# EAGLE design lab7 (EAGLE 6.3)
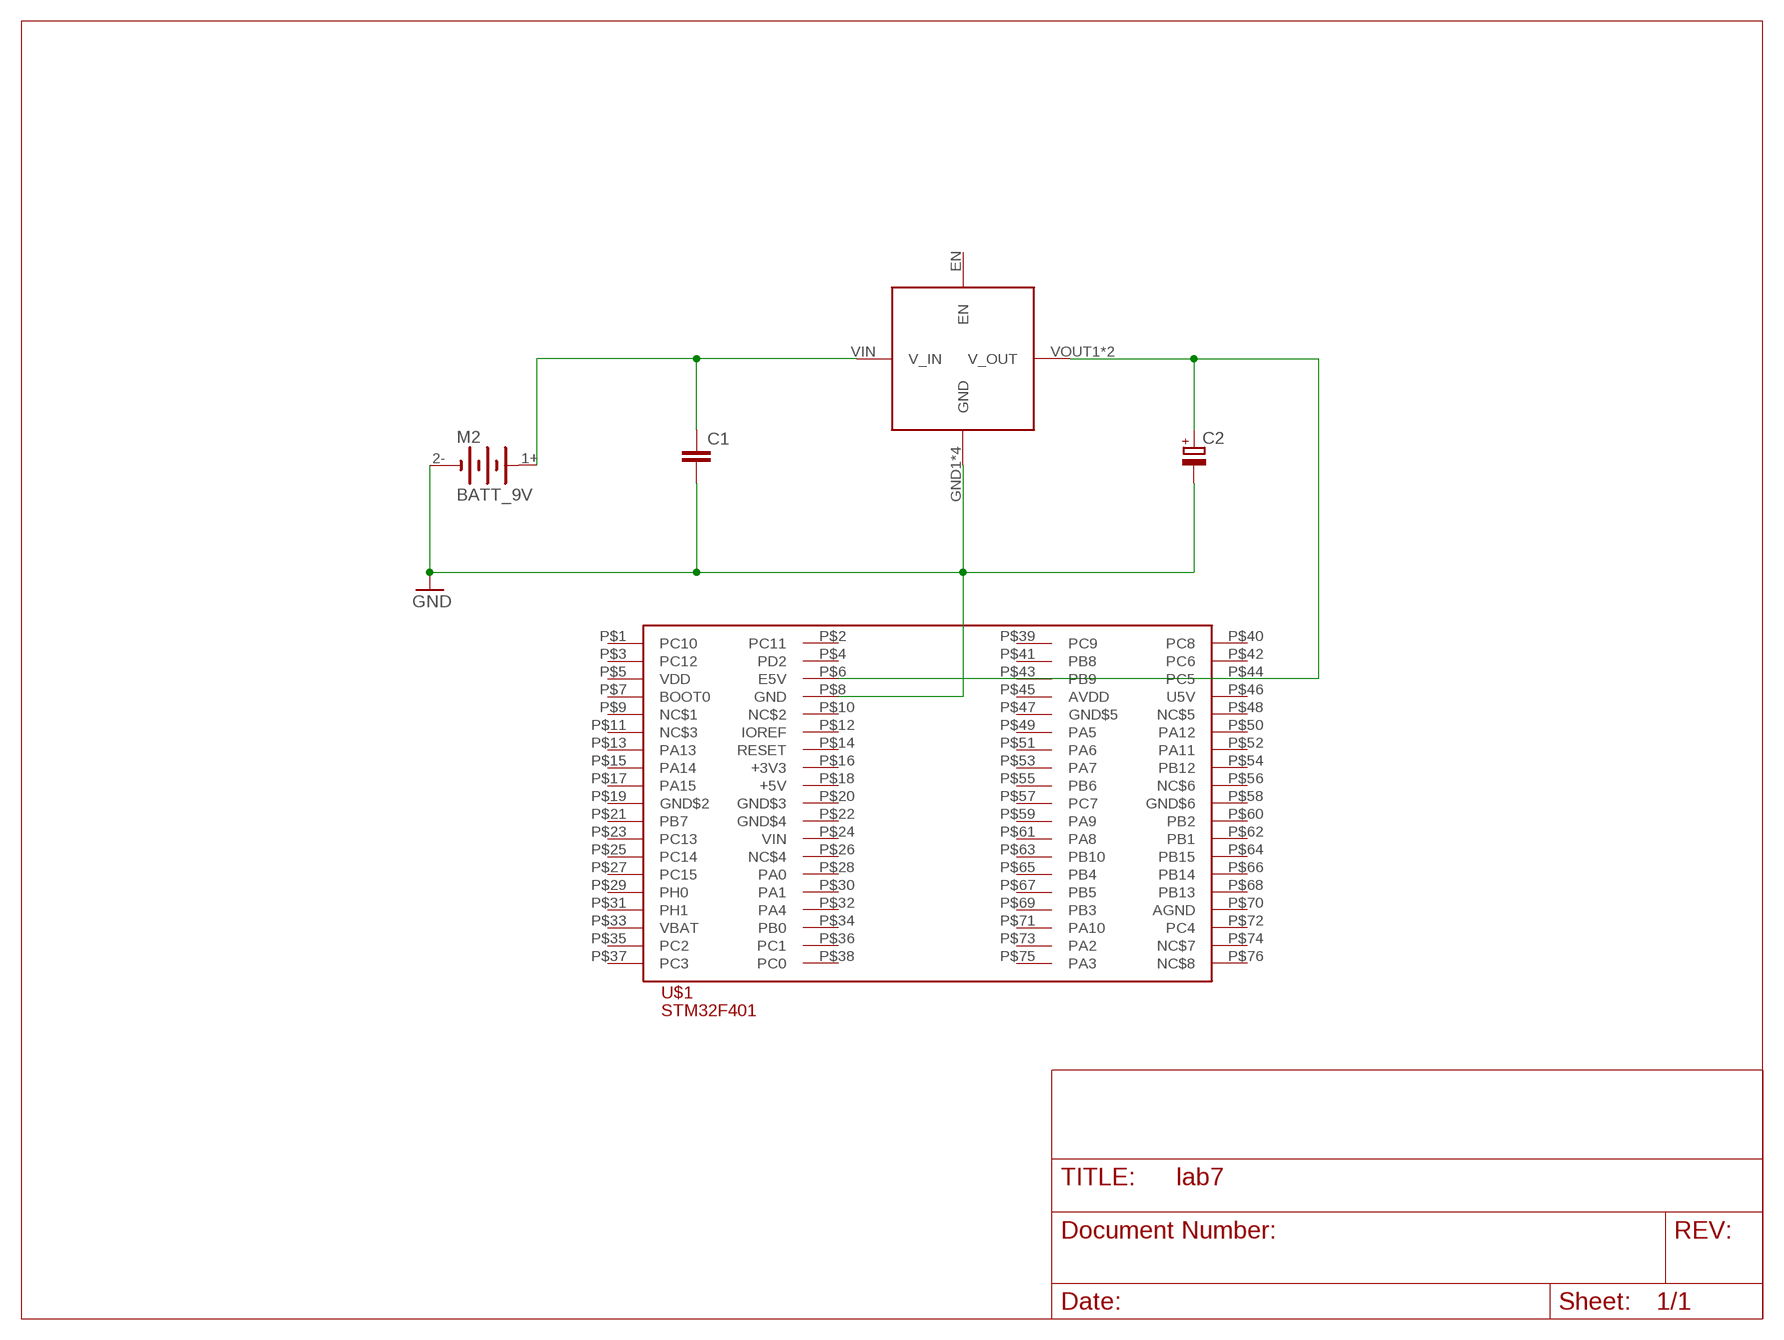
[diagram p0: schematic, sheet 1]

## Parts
C1  C-EU025-025X050  [C025-025X050]
C2  CPOL-EUE3.5-8  [E3,5-8]
M1  PWR_REG  [PWR_REG]
M2  BATT_9V  [BATT_9V]
U$1  STM32401RESTM32P38PKG  [STM32P38]

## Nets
GND: C1.2 C2.- M1.GND1(GND) M1.GND2(GND) M1.GND3(GND) M1.GND4(GND) M2.2-(-) U$1.P$8(GND)
N$2: C1.1 M1.VIN(V_IN) M2.1+(+)
N$3: C2.+ M1.VOUT1(V_OUT) M1.VOUT2(V_OUT) U$1.P$6(E5V)
Unconnected: M1.EN U$1.P$1(PC10) U$1.P$2(PC11) U$1.P$3(PC12) U$1.P$4(PD2) U$1.P$5(VDD) U$1.P$7(BOOT0) U$1.P$9(NC$1) U$1.P$10(NC$2) U$1.P$11(NC$3) U$1.P$12(IOREF) U$1.P$13(PA13) U$1.P$14(RESET) U$1.P$15(PA14) U$1.P$16(+3V3) U$1.P$17(PA15) U$1.P$18(+5V) U$1.P$19(GND$2) U$1.P$20(GND$3) U$1.P$21(PB7) U$1.P$22(GND$4) U$1.P$23(PC13) U$1.P$24(VIN) U$1.P$25(PC14) U$1.P$26(NC$4) U$1.P$27(PC15) U$1.P$28(PA0) U$1.P$29(PH0) U$1.P$30(PA1) U$1.P$31(PH1) U$1.P$32(PA4) U$1.P$33(VBAT) U$1.P$34(PB0) U$1.P$35(PC2) U$1.P$36(PC1) U$1.P$37(PC3) U$1.P$38(PC0) U$1.P$39(PC9) U$1.P$40(PC8) U$1.P$41(PB8) U$1.P$42(PC6) U$1.P$43(PB9) U$1.P$44(PC5) U$1.P$45(AVDD) U$1.P$46(U5V) U$1.P$47(GND$5) U$1.P$48(NC$5) U$1.P$49(PA5) U$1.P$50(PA12) U$1.P$51(PA6) U$1.P$52(PA11) U$1.P$53(PA7) U$1.P$54(PB12) U$1.P$55(PB6) U$1.P$56(NC$6) U$1.P$57(PC7) U$1.P$58(GND$6) U$1.P$59(PA9) U$1.P$60(PB2) U$1.P$61(PA8) U$1.P$62(PB1) U$1.P$63(PB10) U$1.P$64(PB15) U$1.P$65(PB4) U$1.P$66(PB14) U$1.P$67(PB5) U$1.P$68(PB13) U$1.P$69(PB3) U$1.P$70(AGND) U$1.P$71(PA10) U$1.P$72(PC4) U$1.P$73(PA2) U$1.P$74(NC$7) U$1.P$75(PA3) U$1.P$76(NC$8)

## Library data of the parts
C1 = rcl:C-EU: CAPACITOR, European symbol
C2 = rcl:CPOL-EU: POLARIZED CAPACITOR, European symbol
M1 = P442:PWR_REG: Pololu D15V35F5S3
M2 = P442:BATT_9V
U$1 = STM32_lib:STM32401RE

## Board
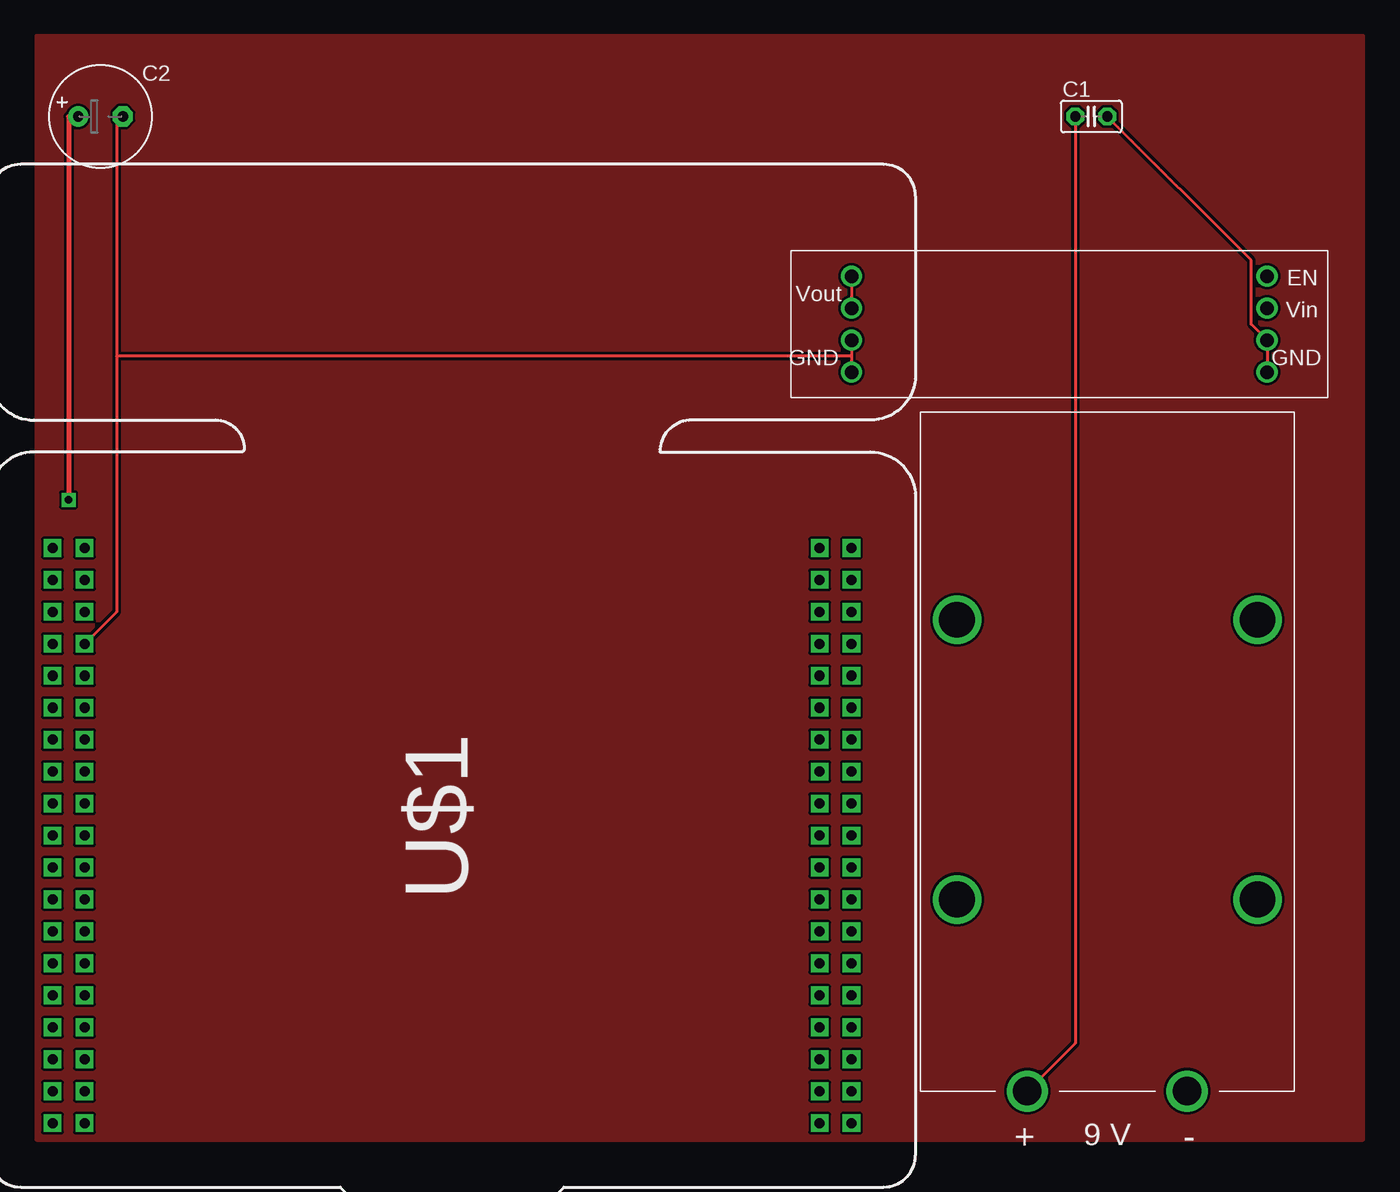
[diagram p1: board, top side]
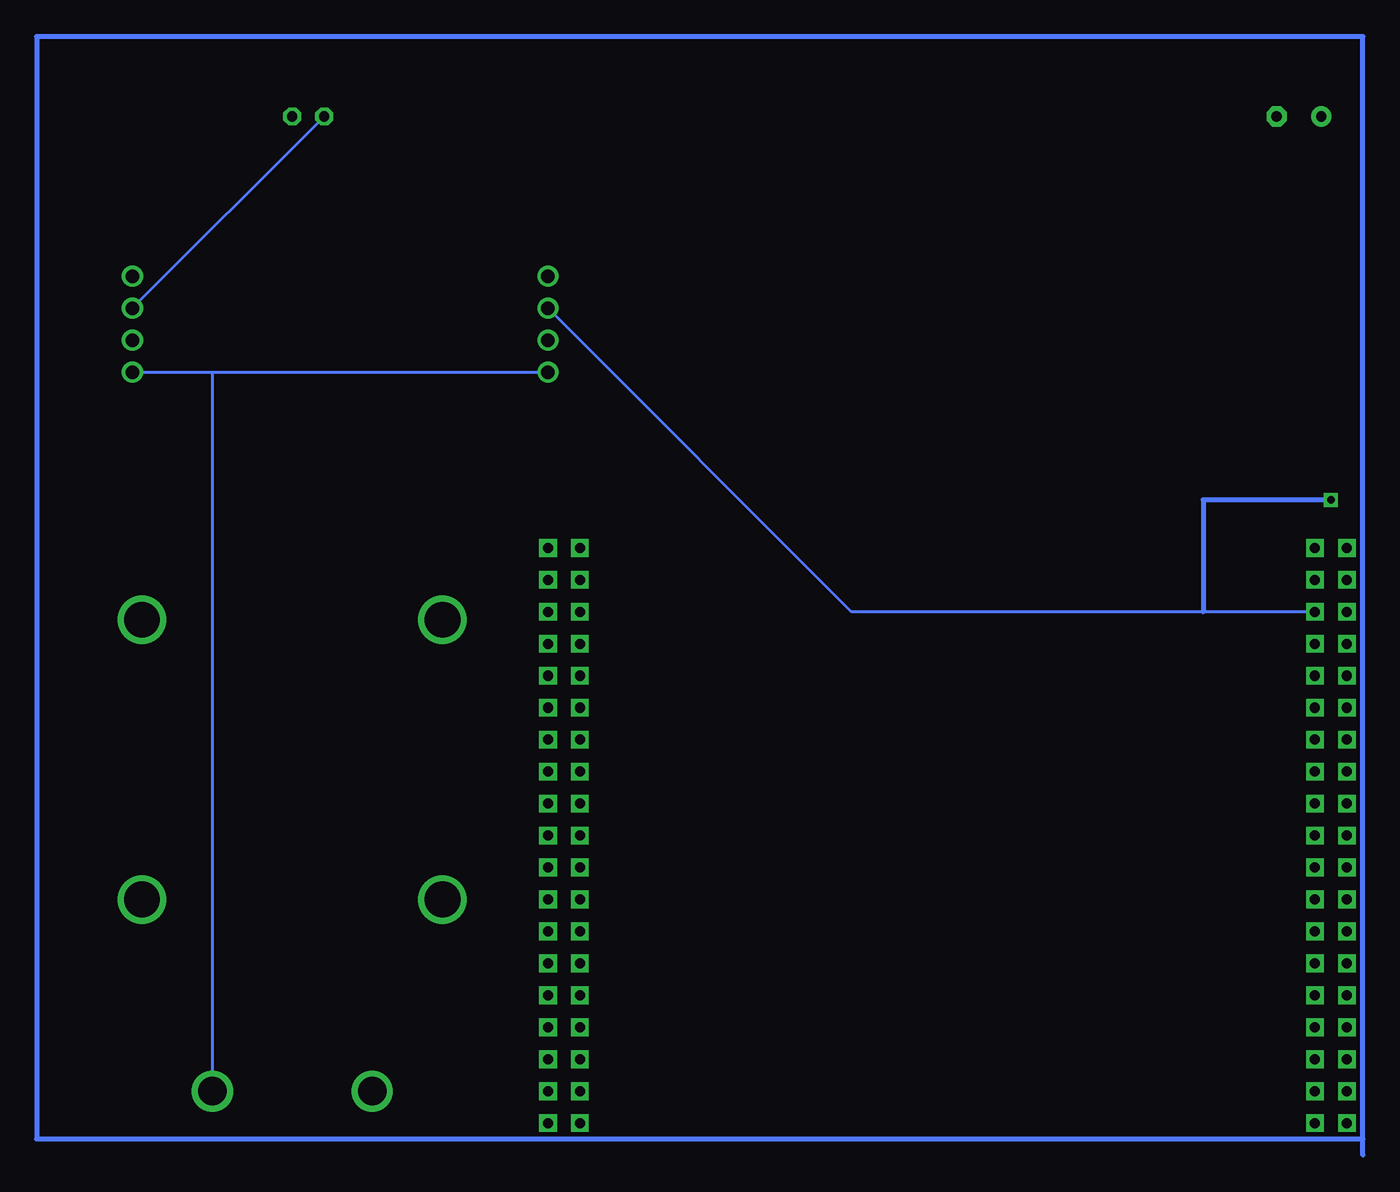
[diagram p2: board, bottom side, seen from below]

No outline drawn. Coordinates in mm, seen from the top.
Copper layers (1*16): Top 0.035mm / dielectric 1.5mm / Bottom 0.035mm
Design rules "SparkFun": minimum track width 8mil, minimum drill 20mil, track to track 8mil, track to pad 8mil, pad to pad 8mil, via to via 8mil, smd to smd 8mil, copper to edge 8mil, drill to drill 8mil, minimum pad ring 12mil, minimum via ring 10mil, stop-mask expansion 4mil, vias tented up to drill 20mil, thermal gap 10mil

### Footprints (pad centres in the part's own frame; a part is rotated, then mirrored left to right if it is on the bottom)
C025-025X050 = drill 0.813 octagon: 1 -1.27,0; 2 1.27,0
E3,5-8 = drill 0.813 pad 1.6: + -1.778,0 | drill 0.813 pad 1.6 octagon: - 1.778,0
PWR_REG = drill 1.067: EN -16.51,-3.81; GND1 -16.51,3.81; GND2 -16.51,1.27; GND3 16.51,3.81; GND4 16.51,1.27; VIN -16.51,-1.27; VOUT1 16.51,-1.27; VOUT2 16.51,-3.81
BATT_9V = drill 2.261: 1+ 0,6.35; 2- 0,-6.35 | drill 2.845: 3 15.24,11.938; 4 15.24,-11.938; 5 37.465,11.938; 6 37.465,-11.938
STM32P38 = drill 0.8 square: P$1 -30.48,1.27; P$2 -27.94,1.27; P$3 -30.48,-1.27; P$4 -27.94,-1.27; P$5 -30.48,-3.81; P$6 -27.94,-3.81; P$7 -30.48,-6.35; P$8 -27.94,-6.35; P$9 -30.48,-8.89; P$10 -27.94,-8.89; P$11 -30.48,-11.43; P$12 -27.94,-11.43; P$13 -30.48,-13.97; P$14 -27.94,-13.97; P$15 -30.48,-16.51; P$16 -27.94,-16.51; P$17 -30.48,-19.05; P$18 -27.94,-19.05; P$19 -30.48,-21.59; P$20 -27.94,-21.59; P$21 -30.48,-24.13; P$22 -27.94,-24.13; P$23 -30.48,-26.67; P$24 -27.94,-26.67; P$25 -30.48,-29.21; P$26 -27.94,-29.21; P$27 -30.48,-31.75; P$28 -27.94,-31.75; P$29 -30.48,-34.29; P$30 -27.94,-34.29; P$31 -30.48,-36.83; P$32 -27.94,-36.83; P$33 -30.48,-39.37; P$34 -27.94,-39.37; P$35 -30.48,-41.91; P$36 -27.94,-41.91; P$37 -30.48,-44.45; P$38 -27.94,-44.45; P$39 30.48,1.27; P$40 33.02,1.27; P$41 30.48,-1.27; P$42 33.02,-1.27; P$43 30.48,-3.81; P$44 33.02,-3.81; P$45 30.48,-6.35; P$46 33.02,-6.35; P$47 30.48,-8.89; P$48 33.02,-8.89; P$49 30.48,-11.43; P$50 33.02,-11.43; P$51 30.48,-13.97; P$52 33.02,-13.97; P$53 30.48,-16.51; P$54 33.02,-16.51; P$55 30.48,-19.05; P$56 33.02,-19.05; P$57 30.48,-21.59; P$58 33.02,-21.59; P$59 30.48,-24.13; P$60 33.02,-24.13; P$61 30.48,-26.67; P$62 33.02,-26.67; P$63 30.48,-29.21; P$64 33.02,-29.21; P$65 30.48,-31.75; P$66 33.02,-31.75; P$67 30.48,-34.29; P$68 33.02,-34.29; P$69 30.48,-36.83; P$70 33.02,-36.83; P$71 30.48,-39.37; P$72 33.02,-39.37; P$73 30.48,-41.91; P$74 33.02,-41.91; P$75 30.48,-44.45; P$76 33.02,-44.45

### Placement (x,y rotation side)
C1  83.82,81.28 0 top
C2  5.08,81.28 0 top
M1  81.28,64.77 180 top
M2  85.09,3.81 90 top
U$1  31.75,45.72 0 top

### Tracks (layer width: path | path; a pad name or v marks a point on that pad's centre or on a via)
GND
  Top 0.254: U$1.P$8 6.35,41.91 6.35,62.23 | 6.35,62.23 6.35,81.28 C2.- | M1.GND4 64.77,62.23 | 64.77,62.23 M1.GND3 | C1.2 96.52,69.85 96.52,64.77 M1.GND2 M1.GND1 | 64.77,62.23 6.35,62.23
  Bottom 0.254: M1.GND1 91.44,60.96 | 91.44,60.96 M1.GND3 | 91.44,60.96 M2.2-
N$1
  Bottom 0.406: 0,-1.27 0,0 | 0,0 0,87.63 105.41,87.63 105.41,0 0,0
N$2
  Top 0.254: M2.1+ 82.55,7.62 C1.1
  Bottom 0.254: M1.VIN C1.1
N$3  (via drill 0.6)
  Top 0.254: M1.VOUT2 M1.VOUT1 | 2.54,81.28 C2.+
  Top 0.406: 2.54,81.28 v2.54,50.8
  Bottom 0.254: M1.VOUT1 40.64,41.91 12.7,41.91 U$1.P$6
  Bottom 0.406: v2.54,50.8 12.7,50.8 12.7,41.91
N$4
  pour Top: 0,0 105.41,0 105.41,87.63 0,87.63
